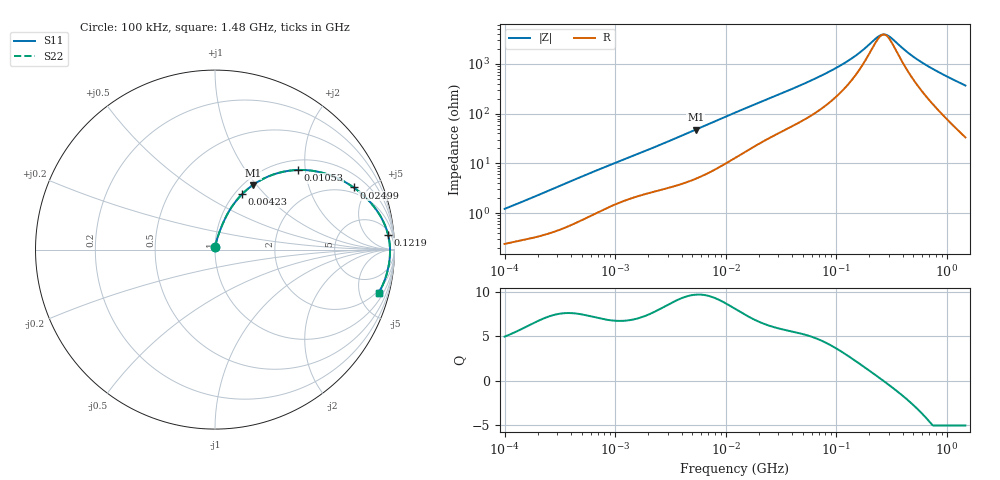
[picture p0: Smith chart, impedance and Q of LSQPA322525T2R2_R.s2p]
! LSQPA322525T2R2_R  S-PARAMETER MODEL  ( General Type )
! Model Generated by TAIYO YUDEN Corporation (http://www.ty-top.com)
! Version 2.0
! TAIYO YUDEN Control No. 100810NF25SB-FKC
! Copyright(c) 2007 TAIYO YUDEN CO.,LTD. All Rights Reserved.
! Product Description (link to TY-COMPAS)
! https://ds.yuden.co.jp/TYCOMPAS/or/detail?pn=LSQPA322525T2R2MR&u=M
! Products Name : Inductors
! Characteristics :
!  Inductance : 2.2 uH , SRF(min) : 190 MHz , DC Resistance(max) : 0.104 Ohm
!  Rated Current : Saturation :2000 mA , Temp Rise : 1130 mA (40 degC)
!  Case Size : 3.2 x 2.5 / 0.126 x 0.098 [mm/inch] , Thickness : 2.5 / 0.098 [mm/inch]
!  (Conditions: Temperature = 25 degC , DC Bias Current/Voltage = 0A / 0V)
! External Node Assignments :
!  1  o---GGG---o  2
! GND o---------o GND
! Frequency Range : 0.1MHz  -  1479.677449MHz  [ 402 STEP ]
# MHz S RI R 50
! Freq[MHz].  S11 Real  S11 Imag  S21 Real  S21 Imag  S12 Real  S12 Imag  S22 Real  S22 Imag
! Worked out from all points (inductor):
!   401 points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, 100 kHz to 1.48 GHz, reference 50 ohm
!   read as one part in series: L = 1.86 uH near 104.9 kHz
!   highest Q = 9.7 at 5.378 MHz (marker M1), where L = 1.41 uH
!   self-resonance near 269.1 MHz
!   S11 on the Smith chart (normalised r, x): 100 kHz: 1.00, +0.02; 4.23 MHz: 1.08, +0.76; 10.53 MHz: 1.21, +1.82; 24.99 MHz: 1.65, +4.03; 121.9 MHz: 8, +20; 1.48 GHz: 1.67, -7.36
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0.1  0.00254 0.0119  0.9975 -0.0119  0.9975 -0.0119  0.00254 0.0119
0.499463  0.01 0.053  0.99 -0.053  0.99 -0.053  0.01 0.053
1.214069  0.0309 0.1142  0.9691 -0.1142  0.9691 -0.1142  0.0309 0.1142
2.494629  0.074 0.2068  0.926 -0.2068  0.926 -0.2068  0.074 0.2068
4.230241  0.1512 0.3091  0.8488 -0.3091  0.8488 -0.3091  0.1512 0.3091
5.377982  0.2103 0.3592  0.7897 -0.3592  0.7897 -0.3592  0.2103 0.3592
7.709045  0.3321 0.4208  0.6679 -0.4208  0.6679 -0.4208  0.3321 0.4208
10.53249  0.4606 0.4435  0.5394 -0.4435  0.5394 -0.4435  0.4606 0.4435
12.45974  0.5316 0.4406  0.4684 -0.4406  0.4684 -0.4406  0.5316 0.4406
24.99459  0.7723 0.3464  0.2277 -0.3464  0.2277 -0.3464  0.7723 0.3464
38.5038  0.8646 0.2643  0.1354 -0.2643  0.1354 -0.2643  0.8646 0.2643
60.75563  0.9241 0.1824  0.0759 -0.1824  0.0759 -0.1824  0.9241 0.1824
89.20582  0.9519 0.1231  0.0481 -0.1231  0.0481 -0.1231  0.9519 0.1231
121.8775  0.9644 0.0825  0.0356 -0.0825  0.0356 -0.0825  0.9644 0.0825
162.5656  0.9709 0.0501  0.0291 -0.0501  0.0291 -0.0501  0.9709 0.0501
244.4898  0.9749 0.00924  0.0251 -0.00924  0.0251 -0.00924  0.9749 0.00924
269.1302  0.9752 -8.51e-06  0.0248 8.51e-06  0.0248 8.51e-06  0.9752 -8.51e-06
303.4516  0.9753 -0.0116  0.0247 0.0116  0.0247 0.0116  0.9753 -0.0116
445.5497  0.9732 -0.0506  0.0268 0.0506  0.0268 0.0506  0.9732 -0.0506
594.2938  0.9687 -0.0841  0.0313 0.0841  0.0313 0.0841  0.9687 -0.0841
915.5007  0.9535 -0.1467  0.0465 0.1467  0.0465 0.1467  0.9535 -0.1467
1479.677  0.9129 -0.2403  0.0871 0.2403  0.0871 0.2403  0.9129 -0.2403
